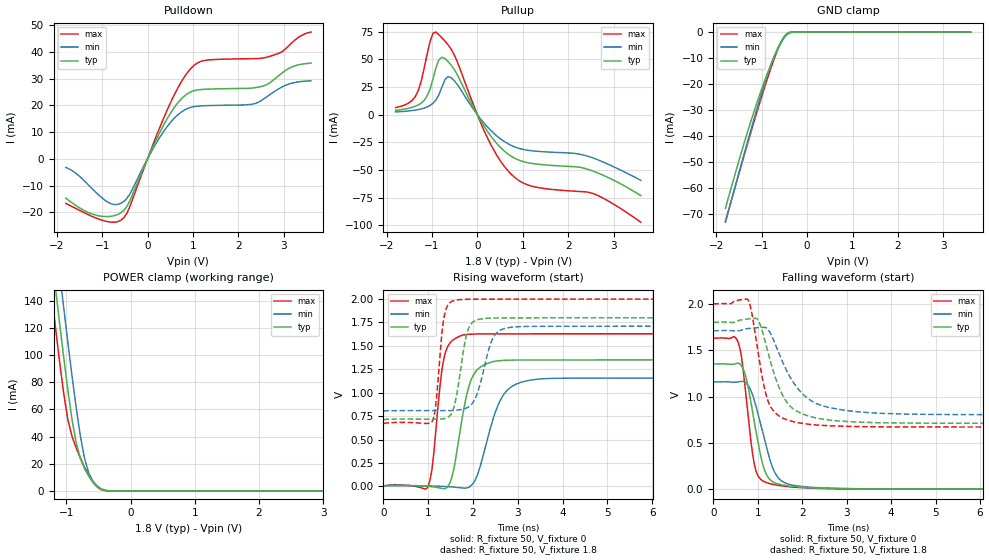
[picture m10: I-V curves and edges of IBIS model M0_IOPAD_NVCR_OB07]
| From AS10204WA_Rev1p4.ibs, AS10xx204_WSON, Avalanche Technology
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[Model] M0_IOPAD_NVCR_OB07
Model_type I/O
Enable   Active-High
Vinl  =  0.54
Vinh  =  1.26
Vmeas =  0.9
Cref  =  30e-12
| Capacitance  typ   min   max
C_comp   3.869840e-12   3.575244e-12   4.208825e-12
| Variables   typ   min   max
[GND Clamp Reference]   0   0   0
[POWER Clamp Reference]   1.8   1.71   2
[Pulldown Reference]   0   0   0
[Pullup Reference]   1.8   1.71   2
[Temperature Range]   25   105   -40
[Voltage Range]   1.8   1.71   2
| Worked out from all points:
|   slope of the pulldown table from 0 to 0.27 V, typ, clamps not added: 27.4 ohm
|   slope of the pullup table from 0 to 0.27 V, typ, clamps not added: 15.2 ohm
|   GND clamp passes 1 mA (typ) near -0.46 V on its own axis
|   POWER clamp passes 1 mA (typ) near -0.44 V on its own axis
|   falling waveform, R_fixture 50, V_fixture 0: 20-80 % time 318ps typ, 393ps min, 234ps max; typ from 1.35 V to 0 V
|   falling waveform, R_fixture 50, V_fixture 1.8: 20-80 % time 494ps typ, 688ps min, 317ps max; typ from 1.8 V to 0.711 V
|   rising waveform, R_fixture 50, V_fixture 0: 20-80 % time 313ps typ, 445ps min, 208ps max; typ from 0 V to 1.35 V
|   rising waveform, R_fixture 50, V_fixture 1.8: 20-80 % time 222ps typ, 308ps min, 147ps max; typ from 0.711 V to 1.8 V
[GND Clamp]
| Voltage   I(typ)   I(min)   I(max)
-1.8V     -67.84mA   -73.19mA   -72.81mA
-1.499V   -49.26mA   -53.93mA   -54.28mA
-1.303V   -37.87mA   -41.64mA   -42.4mA
-1.108V   -27.29mA   -29.68mA   -30.84mA
-912.4mV  -17.6mA    -18.46mA   -19.84mA
-782.1mV  -11.7mA    -11.87mA   -13.01mA
-651.7mV  -6.447mA   -6.494mA   -6.896mA
-521.4mV  -2.255mA   -2.526mA   -2.141mA
-456.2mV  -849.3uA   -1.156mA   -679.4uA
-391mV    -172uA     -356.5uA   -88.88uA
-260.7mV  -2.088uA   -12.98uA   -254.3nA
3.6V      0A         0A         0A
[POWER Clamp]
| Voltage   I(typ)   I(min)   I(max)
-1.8V     419.8mA    456.6mA    390.9mA
-1.238V   178mA      215.7mA    148.4mA
-1.173V   151mA      188.6mA    121.7mA
-1.108V   124.5mA    161.8mA    96mA
-1.043V   98.85mA    135.4mA    72.14mA
-977.6mV  74.56mA    109.6mA    52.56mA
-912.4mV  52.76mA    84.78mA    40.16mA
-847.2mV  35.48mA    61.36mA    31.71mA
-716.9mV  16.42mA    23.91mA    17.31mA
-651.7mV  10.9mA     13.27mA    11.28mA
-456.2mV  1.168mA    1.554mA    921.1uA
3.6V      0A         0A         0A
[Pulldown]
| Voltage   I(typ)   I(min)   I(max)
-1.8V     -14.7mA    -3.206mA   -16.67mA
-1.173V   -20.9mA    -11.95mA   -21.89mA
-847.2mV  -21.57mA   -16.46mA   -23.58mA
-586.6mV  -20.2mA    -16.62mA   -22.98mA
-391mV    -15.81mA   -13.23mA   -17.94mA
434.5mV   15.06mA    12.09mA    18.3mA
993.1mV   25.32mA    19.42mA    34.48mA
1.303V    26.05mA    19.9mA     36.91mA
2.283V    26.44mA    20.38mA    37.46mA
2.697V    28.46mA    24.05mA    38.33mA
3.179V    34.35mA    28.3mA     43.4mA
3.6V      35.79mA    29.21mA    47.41mA
[Pullup]
| Voltage   I(typ)   I(min)   I(max)
-1.8V     3.929mA    2.431mA    6.328mA
-1.369V   7.544mA    4.11mA     16.15mA
-1.108V   16.63mA    6.881mA    54.24mA
-977.6mV  32.17mA    10.22mA    73.42mA
-912.4mV  42.21mA    13.23mA    74.52mA
-782.1mV  51.81mA    24.67mA    69.4mA
-586.6mV  45.15mA    33.59mA    59.67mA
248.3mV   -16.56mA   -12.19mA   -23.05mA
744.8mV   -37.5mA    -27.71mA   -53.73mA
1.241V    -44.25mA   -32.78mA   -64.98mA
2.559V    -51.13mA   -39.24mA   -71.32mA
3.6V      -73.01mA   -59.25mA   -97.05mA
[Ramp]
dV/dt_r   0.810285/0.312866n  0.694157/0.445387n  0.977638/0.208143n
dV/dt_f   0.653673/0.494413n  0.544179/0.687513n  0.797534/0.316527n
R_load = 50
[Falling Waveform]
R_fixture = 50
V_fixture = 0
V_fixture_min = 0
V_fixture_max = 0
| Time   V(typ)   V(min)   V(max)
0s        1.35V      1.157V     1.629V
542ps     1.36V      1.155V     1.606V
629.8ps   1.336V     1.163V     1.446V
734.7ps   1.213V     1.149V     1.022V
866.2ps   887.8mV    1.043V     448.9mV
949.7ps   657.2mV    918.5mV    218.5mV
1.175ns   179.9mV    501.2mV    75.52mV
1.514ns   49.17mV    98.37mV    37mV
3.559ns   1.954mV    3.127mV    1.261mV
21.88ns   541.3nV    1.045uV    488.8nV
[Falling Waveform]
R_fixture = 50
V_fixture = 1.8
V_fixture_min = 1.71
V_fixture_max = 2
| Time   V(typ)   V(min)   V(max)
0s        1.8V       1.71V      2V
777.8ps   1.837V     1.733V     2.047V
868.5ps   1.841V     1.738V     1.899V
1.028ns   1.808V     1.744V     1.417V
1.269ns   1.412V     1.698V     909mV
1.651ns   940.8mV    1.28V      749.7mV
2.09ns    797.8mV    993.8mV    703.5mV
2.77ns    738.1mV    866.7mV    681.2mV
4.192ns   714.2mV    812.1mV    671.9mV
21.88ns   710.5mV    803mV      670.8mV
[Rising Waveform]
R_fixture = 50
V_fixture = 0
V_fixture_min = 0
V_fixture_max = 0
| Time   V(typ)   V(min)   V(max)
0s        87.47nV    395.4nV    147.8nV
983.1ps   758.9uV    4.754mV    -13.23mV
1.089ns   -4.069mV   3.676mV    198.8mV
1.357ns   -25.09mV   -1.067mV   1.378V
1.535ns   106.6mV    -6.015mV   1.555V
1.829ns   908mV      -19.66mV   1.62V
2.084ns   1.239V     102.9mV    1.627V
2.693ns   1.345V     985.1mV    1.629V
3.46ns    1.35V      1.145V     1.629V
21.88ns   1.35V      1.157V     1.629V
[Rising Waveform]
R_fixture = 50
V_fixture = 1.8
V_fixture_min = 1.71
V_fixture_max = 2
| Time   V(typ)   V(min)   V(max)
0s        710.5mV    803mV      670.8mV
1.098ns   715.4mV    808.5mV    701.2mV
1.175ns   715.6mV    808.1mV    895.6mV
1.359ns   723.6mV    808.2mV    1.818V
1.644ns   999.8mV    813.3mV    1.991V
1.828ns   1.56V      832mV      1.997V
1.945ns   1.727V     864.7mV    1.998V
2.442ns   1.797V     1.578V     1.999V
2.869ns   1.799V     1.7V       1.999V
21.88ns   1.8V       1.71V      2V
